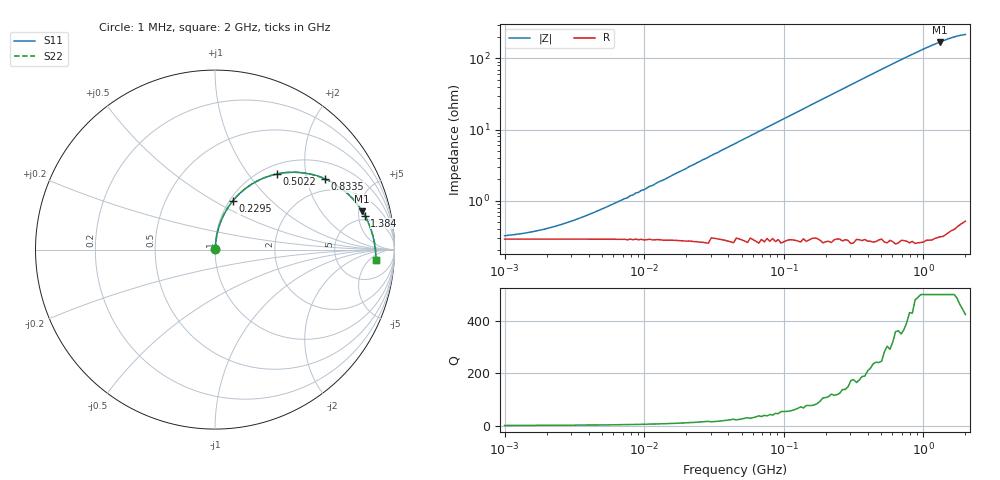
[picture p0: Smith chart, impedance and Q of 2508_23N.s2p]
# MHz S MA R 50
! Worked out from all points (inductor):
!   166 points, 1 MHz to 2 GHz, reference 50 ohm
!   read as one part in series: L = 22.6 nH near 6.313 MHz
!   highest Q = 552 at 1.321 GHz (marker M1), where L = 20.7 nH
!   S11 on the Smith chart (normalised r, x): 1 MHz: 1.01, +0.00; 229.5 MHz: 1.04, +0.61; 502.2 MHz: 1.16, +1.40; 833.5 MHz: 1.54, +2.58; 1.384 GHz: 4.24, +6.00; 2 GHz: 14, -8
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1  0.003039 25.4  0.997 -0.1  0.997 -0.1  0.00304 25.5
1.906  0.003708 42.1  0.997 -0.2  0.997 -0.2  0.00371 42.2
3.632  0.00549 59.7  0.997 -0.3  0.997 -0.3  0.005494 59.7
7.591  0.01 73.9  0.997 -0.7  0.997 -0.7  0.01 73.9
7.948  0.011 74.5  0.997 -0.7  0.997 -0.7  0.011 74.6
10.007  0.013 77.3  0.997 -0.9  0.997 -0.9  0.013 77.3
10.973  0.015 78.2  0.997 -1.0  0.997 -1.0  0.015 78.2
11.49  0.015 78.7  0.997 -1.0  0.997 -1.0  0.015 78.7
12.599  0.017 79.5  0.997 -1.1  0.997 -1.1  0.017 79.5
13.193  0.017 79.8  0.997 -1.1  0.997 -1.1  0.018 79.8
13.815  0.018 80.2  0.997 -1.2  0.997 -1.2  0.018 80.2
45.763  0.06 83.4  0.995 -4.0  0.995 -4.0  0.06 83.4
91.33  0.119 80.8  0.99 -7.9  0.99 -7.9  0.119 80.8
166.224  0.212 75.0  0.974 -14.3  0.974 -14.3  0.213 75.0
229.476  0.287 70.0  0.955 -19.5  0.955 -19.5  0.288 70.0
347.37  0.413 61.1  0.908 -28.6  0.908 -28.6  0.413 61.1
502.161  0.546 50.6  0.835 -39.2  0.835 -39.2  0.546 50.6
576.582  0.598 46.0  0.799 -43.8  0.799 -43.8  0.598 46.0
833.511  0.728 32.8  0.683 -57.1  0.683 -57.1  0.729 32.8
1321.216  0.847 14.7  0.529 -75.2  0.529 -75.2  0.848 14.7
1383.503  0.856 12.8  0.515 -77.1  0.515 -77.1  0.857 12.8
2000  0.898 -3.7  0.435 -93.6  0.435 -93.6  0.899 -3.7
